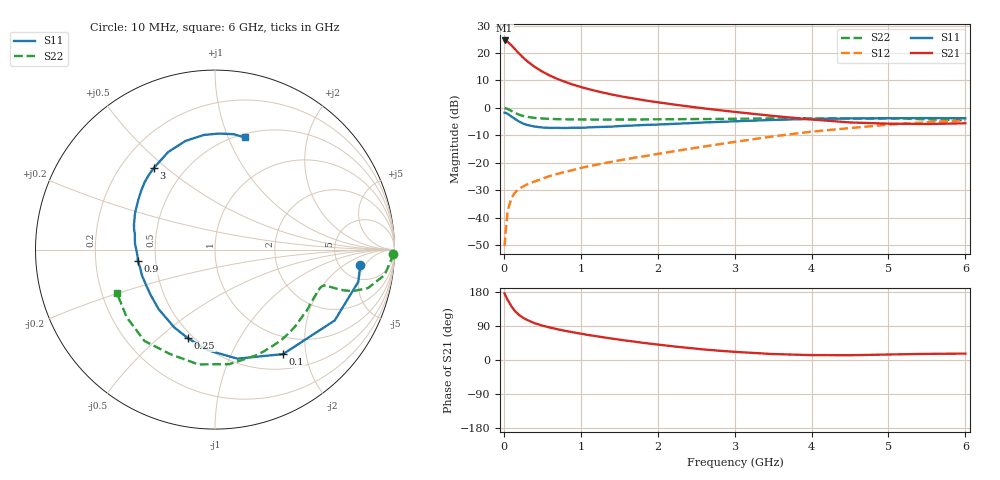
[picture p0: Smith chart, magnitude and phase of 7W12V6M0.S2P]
! Infineon Technologies  Discrete & RF Semiconductors
! BFS17W
! Si NPN RF Bipolar Junction Transistor in SOT323
! VCE = 12 V  IC = 6 mA
! Common Emitter S-Parameters:  August  1999
# GHz  S  MA  R  50
!  f  S11  S21  S12  S22
! GHz  MAG  ANG  MAG  ANG  MAG  ANG  MAG  ANG
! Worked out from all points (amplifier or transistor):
!   36 points, 10 MHz to 6 GHz, reference 50 ohm
!   highest |S21| = 24.6 dB at 10 MHz (marker M1)
!   |S21| within 3 dB of that: start of sweep to 139.1 MHz
!   unconditionally stable (mu >= 1): 565.7 MHz to 2.213 GHz; 5.499 GHz to end of sweep
!   at 250 MHz: K = 0.63, MSG = 23.5 dB, |S12| = -28.7 dB
!   at 1.4 GHz: K = 1.18, MAG = 9.7 dB, |S12| = -19.7 dB
!   at 6 GHz: K = 1.04, MAG = -1.7 dB, |S12| = -4.5 dB
!   S11 on the Smith chart (normalised r, x): 10 MHz: 7.66, -4.00; 100 MHz: 0.71, -1.61; 250 MHz: 0.47, -0.63; 900 MHz: 0.40, -0.06; 3 GHz: 0.34, +0.45; 6 GHz: 0.54, +1.15
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0.01  0.8143 -6.2  16.98 175.6  0.003 81.6  0.9943 -1.3
0.02  0.8182 -12.7  16.88 170.9  0.0048 83.5  0.9818 -3.6
0.05  0.7751 -30.6  15.99 158.4  0.0133 77.8  0.9555 -8.5
0.1  0.6948 -56.9  13.78 141.2  0.0229 64.7  0.8792 -14.1
0.15  0.6203 -78.4  11.57 127.9  0.029 57.8  0.8037 -16.7
0.2  0.5616 -94.3  9.744 118.6  0.0335 55.4  0.7504 -17.6
0.25  0.5162 -107.0  8.278 111.5  0.0368 52.7  0.7125 -17.8
0.3  0.4894 -117.6  7.17 105.9  0.04 53.1  0.6879 -17.9
0.4  0.4567 -133.5  5.611 97.2  0.0454 54.0  0.6555 -18.0
0.5  0.4387 -145.0  4.589 90.9  0.0509 55.9  0.64 -18.2
0.6  0.4315 -153.5  3.867 85.6  0.0574 57.5  0.6296 -19.0
0.7  0.4317 -160.5  3.359 81.1  0.0626 59.7  0.6228 -20.1
0.9  0.4347 -171.7  2.652 73.1  0.0735 62.2  0.6147 -22.8
1.1  0.4396 179.4  2.202 65.9  0.0863 64.4  0.613 -26.1
1.3  0.4507 172.1  1.886 59.7  0.098 66.6  0.611 -29.8
1.6  0.4728 162.7  1.553 50.9  0.1163 68.8  0.6124 -35.8
2.2  0.5099 146.8  1.157 36.1  0.1606 72.5  0.6216 -49.3
3  0.5684 126.8  0.845 21.5  0.2394 72.9  0.6319 -69.0
3.5  0.6032 115.6  0.713 15.7  0.302 70.2  0.643 -82.9
4.5  0.6418 95.5  0.542 12.6  0.4283 59.0  0.6335 -113.2
5.5  0.6513 80.8  0.508 16.2  0.5467 45.5  0.6197 -142.6
6  0.6466 75.1  0.523 16.9  0.5934 38.7  0.5975 -155.9
